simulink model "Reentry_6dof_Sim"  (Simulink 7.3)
settings: Solver=ode45  StartTime=0.0  StopTime=1943  FixedStep=0.01
InitFcn:
  | init
StopFcn:
  | pl
  | save_traj
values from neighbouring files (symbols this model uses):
  d2r = pi/180    (= 0.0174532925199)    [init.m]    (also in pl.m; robust.m)
  h0 = 250000.0    (= 250000)    [init.m]
  mass = 528.0    (= 528)    [init.m]
  r2d = 180/pi    (= 57.2957795131)    [init.m]    (also in pl.m; robust.m)
  sp = 15    [init.m]
  x0 = [0 0 -2 -2 0 0 18 0 0 0]'*d2r    [init.m]
  x_cg = -17.04    [init.m]
  x_ref = -16.2    [init.m]
  y_cg = 0    [init.m]
  z_cg = -2.03    [init.m]
  z_ref = -2.1    [init.m]
undefined symbols (not defined in the file or in its folder): Cl, Cld1, Cld2, Cld3, Cld4, Cld5, Cld6, Cld7, Cm, Cmd1, Cmd2, Cmd3, Cmd4, Cmd5, Cmd6, Cmd7, Cn, Cnd1, Cnd2, Cnd3, Cnd4, Cnd5, Cnd6, Cnd7, CX, CXd1, CXd2, CXd3, CXd4, CXd5, CXd6, CXd7, CY, CYd1, CYd2, CYd3, CYd4, CYd5, CYd6, CYd7, CZ, CZd1, CZd2, CZd3, CZd4, CZd5, CZd6, CZd7, ft, HDBK, km, Lateral_FCS, MIL, Pitch_FCS, sigbuilder_block
libraries: aerolibasang x3, aerolib6dof2 x1, aerolibconvert2 x1, aerolibatmos2 x1, aerolibgravity2 x1, aerolibadyn x1
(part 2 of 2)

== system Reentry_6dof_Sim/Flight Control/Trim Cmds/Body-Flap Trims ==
  Demux : Demux  Tag=STV Demux
  FromWs : FromWorkspace  Tag=STV FromWs  VariableName=tuvar  SampleTime=0  SigBuilderData=DataTag6  VnvData=DataTag7
  Up-Left BF : Outport  Tag=STV Outport
  Up Right BF : Outport  Tag=STV Outport  Port=2
  Lo-Left BF : Outport  Tag=STV Outport  Port=3
  Lo-Right BF : Outport  Tag=STV Outport  Port=4
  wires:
  FromWs/1 -> Demux/1
  Demux/1 -> Up-Left BF/1
  Demux/2 -> Up Right BF/1
  Demux/3 -> Lo-Left BF/1
  Demux/4 -> Lo-Right BF/1

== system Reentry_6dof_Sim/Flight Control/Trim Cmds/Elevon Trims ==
  Demux : Demux  Tag=STV Demux  Outputs=2
  FromWs : FromWorkspace  Tag=STV FromWs  VariableName=tuvar  SampleTime=0  SigBuilderData=DataTag8  VnvData=DataTag9
  Left Elev : Outport  Tag=STV Outport
  Right Elev : Outport  Tag=STV Outport  Port=2
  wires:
  FromWs/1 -> Demux/1
  Demux/1 -> Left Elev/1
  Demux/2 -> Right Elev/1

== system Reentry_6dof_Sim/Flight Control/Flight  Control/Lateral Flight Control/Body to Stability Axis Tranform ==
  note: Body to Stability Axes Transformation
  p_b : Inport  OutDataType=sfix(16)  OutScaling=2^0
  r_b : Inport  Port=2  OutDataType=sfix(16)  OutScaling=2^0
  Cos : Subsystem
  "Cos " : Subsystem
  Sin : Subsystem
  "Sin " : Subsystem
  Sum1 : Sum  Inputs=+|+  OutDataType=sfix(16)  OutScaling=2^0
  Sum2 : Sum  Inputs=+|-  OutDataType=sfix(16)  OutScaling=2^0
  p_s : Outport  OutDataType=sfix(16)  OutScaling=2^0
  r_s : Outport  Port=2  OutDataType=sfix(16)  OutScaling=2^0
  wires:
  Sum1/1 -> p_s/1
  Sum2/1 -> r_s/1
  p_b/1 -> Cos/2(in), "Sin "/2(in)
  r_b/1 -> Sin/2(in), "Cos "/2(in)
  Sin/1(sa) -> Sum1/2
  "Cos "/1(ca) -> Sum2/1
  "Sin "/1(sa) -> Sum2/2
  Cos/1(ca) -> Sum1/1
  [alfa] -> Cos/1(alf), Sin/1(alf), "Cos "/1(alf), "Sin "/1(alf)

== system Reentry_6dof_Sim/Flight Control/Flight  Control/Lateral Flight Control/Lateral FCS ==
  ae : Inport
  xlat : Inport  Port=2
  Demux2 : Demux  Outputs=[7,2]
  Lateral_FCS.m : MATLABFcn  MATLABFcn=Lateral_FCS( u(1:5), u(6), u(7) )  OutputDimensions=9
  Mux3 : Mux  Inputs=[5, 1,1]
  a,q : Scope
  delta : Outport
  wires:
  Lateral_FCS.m/1 -> Demux2/1
  Demux2/2 -> a,q/1
  Mux3/1 -> Lateral_FCS.m/1
  [Mach] -> Mux3/3
  ae/1 -> Mux3/2
  xlat/1 -> Mux3/1
  Demux2/1 -> delta/1

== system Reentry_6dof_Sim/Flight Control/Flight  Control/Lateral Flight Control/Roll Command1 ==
  Demux : Demux  Tag=STV Demux  Outputs=1
  FromWs : FromWorkspace  Tag=STV FromWs  VariableName=tuvar  SampleTime=0  SigBuilderData=DataTag2  VnvData=DataTag3
  Phi_cmd : Outport  Tag=STV Outport
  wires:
  FromWs/1 -> Demux/1
  Demux/1 -> Phi_cmd/1

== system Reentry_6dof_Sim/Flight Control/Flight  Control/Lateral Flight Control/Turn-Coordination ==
  note: Turn Coordination Rff = (g/V0)*sin(phi)
  phi : Inport
  Divide : Product  Inputs=**/  OutDataType=fixdt(1, 16)  OutScaling=2^-10
  g : Constant  Value=-32.174  OutDataType=fixdt(1, 16)  OutScaling=2^0
  sin : Trigonometry
  Rff : Outport
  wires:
  [V0] -> Divide/3
  sin/1 -> Divide/1
  phi/1 -> sin/1
  Divide/1 -> Rff/1
  g/1 -> Divide/2

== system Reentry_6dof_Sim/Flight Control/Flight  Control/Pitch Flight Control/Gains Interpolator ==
  note: Flight Control Gains Interpolation
  note: alpha - alpha_cmd
  note: State-Feedback Vectors
  xq : Inport
  alferr : Inport  Port=2
  Demux2 : Demux  Outputs=[7,2]
  Mux3 : Mux  Inputs=[7, 1,1]
  Pitch_FCS.m : MATLABFcn  MATLABFcn=Pitch_FCS( u(1:7), u(8), u(9) )  OutputDimensions=9
  a,q : Scope
  delt2 : Scope
  Deltas : Outport
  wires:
  Pitch_FCS.m/1 -> Demux2/1
  Demux2/1 -> Deltas/1, delt2/1
  Demux2/2 -> a,q/1
  Mux3/1 -> Pitch_FCS.m/1
  xq/1 -> Mux3/1
  alferr/1 -> Mux3/2
  [Mach] -> Mux3/3

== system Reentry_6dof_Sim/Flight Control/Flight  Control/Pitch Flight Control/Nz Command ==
  Demux : Demux  Tag=STV Demux  Outputs=1
  FromWs : FromWorkspace  Tag=STV FromWs  VariableName=tuvar  SampleTime=0  SigBuilderData=DataTag4  VnvData=DataTag5
  Nz_cmd : Outport  Tag=STV Outport
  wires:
  FromWs/1 -> Demux/1
  Demux/1 -> Nz_cmd/1

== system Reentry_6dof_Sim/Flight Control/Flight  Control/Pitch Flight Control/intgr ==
  ge : Inport
  Switch : Switch  Threshold=4  OutDataType=fixdt(1, 16)  OutScaling=2^0
  gamin : Integrator  UpperSaturationLimit=20  LowerSaturationLimit=-20
  gamint : Scope
  gamint1 : Scope
  gr : Ground
  gi : Outport
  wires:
  Switch/1 -> gamin/1
  gr/1 -> Switch/1
  [Mach] -> Switch/2
  ge/1 -> Switch/3, gamint1/1
  gamin/1 -> gi/1, gamint/1  "gamin"

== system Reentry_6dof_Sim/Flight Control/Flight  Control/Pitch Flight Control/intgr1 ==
  nze : Inport
  Switch : Switch  Threshold=17  OutDataType=fixdt(1, 16)  OutScaling=2^0
  gamin : Integrator  UpperSaturationLimit=20  LowerSaturationLimit=-20
  gr : Ground
  nzeint : Scope
  nzi : Outport
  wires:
  Switch/1 -> gamin/1
  gr/1 -> Switch/1
  [Mach] -> Switch/2
  nze/1 -> Switch/3
  gamin/1 -> nzi/1, nzeint/1  "gamin"

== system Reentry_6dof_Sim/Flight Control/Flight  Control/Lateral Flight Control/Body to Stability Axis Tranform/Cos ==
  alf : Inport
  in : Inport  Port=2  OutDataType=sfix(16)  OutScaling=2^0
  Product : Product  OutDataType=fixdt(1, 16)  OutScaling=2^0
  cos : Trigonometry  Operator=cos
  ca : Outport
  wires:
  cos/1 -> Product/1
  in/1 -> Product/2
  alf/1 -> cos/1
  Product/1 -> ca/1

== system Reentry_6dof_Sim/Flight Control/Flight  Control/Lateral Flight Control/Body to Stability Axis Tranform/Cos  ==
  alf : Inport
  in : Inport  Port=2  OutDataType=sfix(16)  OutScaling=2^0
  Product : Product  OutDataType=fixdt(1, 16)  OutScaling=2^0
  cos : Trigonometry  Operator=cos
  ca : Outport
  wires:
  cos/1 -> Product/1
  in/1 -> Product/2
  alf/1 -> cos/1
  Product/1 -> ca/1

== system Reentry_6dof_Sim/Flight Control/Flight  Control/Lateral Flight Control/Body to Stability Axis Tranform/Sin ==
  alf : Inport
  in : Inport  Port=2  OutDataType=sfix(16)  OutScaling=2^0
  Product : Product  OutDataType=fixdt(1, 16)  OutScaling=2^0
  sin : Trigonometry
  sa : Outport
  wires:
  sin/1 -> Product/1
  in/1 -> Product/2
  alf/1 -> sin/1
  Product/1 -> sa/1

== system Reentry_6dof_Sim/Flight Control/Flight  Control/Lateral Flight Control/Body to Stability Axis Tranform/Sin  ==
  alf : Inport
  in : Inport  Port=2  OutDataType=sfix(16)  OutScaling=2^0
  Product : Product  OutDataType=fixdt(1, 16)  OutScaling=2^0
  sin : Trigonometry
  sa : Outport
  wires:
  sin/1 -> Product/1
  in/1 -> Product/2
  alf/1 -> sin/1
  Product/1 -> sa/1
